PROGRAM SWProducts
(*SwenChen 2016.7.21 编辑为ＴＣ３*)
VAR
	fb_RecipeManCommands: 		RecipeManCommands;
	fbDirectoryCopy:			FB_DirectoryCopy;
	fbFileDelete:				FB_FileDelete;
	fbEnumFindFileEntry:		FB_EnumFindFileEntry;
	fbCreateDir:				FB_CreateDir;
	F_TRIGLOAD: 			F_TRIG;
	F_TRIGSave: 			F_TRIG;
	F_TRIGLOADFromUSB: 		F_TRIG;
	F_TRIGSaveToUSB: 		F_TRIG;
	F_TRIGDel: 				F_TRIG;
	F_TRIGYes: 				F_TRIG;
	F_TRIGNo: 				F_TRIG;
	TOF_File_load: 			TOF;
	stepLoad: 				INT;
	stepSave: 				INT;
	stepLoadFromUSB: 		INT;
	stepSaveToUSB: 			INT;
	stepDel: 					INT;
	stepInit: 					INT:=0;
	i:						INT;
	n: 						INT;
	j: 						INT;
	TimeCount:				INT;
	bInitState:				BOOL;
	bInit: 					BOOL:=TRUE;
	bInit_fbWritePersistentData: BOOL := TRUE;

	iLastSelIndex:			INT;
	TON_AutoReset: TON;
	DeviceNum: INT := 1;
	sDevice: STRING(INT#12);
	TON_WaitDone: TON;
END_VAR

DeviceNum:=1;	(*XP/CE操作系统选择*)

IF vbtLoad OR vbtSave THEN
	CASE DeviceNum OF
		1:(*xp*)
			sDevice:='C:\Products\';//不建议修改保存目录，其他地方也可能要改的
		2:(*usb*)
			;
		3:(*ce*)
			sDevice:='\Hard Disk\Products\';//不建议修改保存目录，其他地方也可能要改的
	END_CASE;
END_IF


IF NOT bInitState THEN
	Init();
ELSE
	IF ShowDiag THEN
		;//FB_FreePluse1s(tPluseCyle:=t#1s);
	END_IF
	F_TRIGYes(CLK:=vbtYes);
	F_TRIGNo(CLK:=vbtNo);
	HMISelect();
	ButtonDelet();
	ButtonLoad();
	ButtonSave();
	ButtonLoadFromUSB();
	ButtonSaveToUSB();
	ReflashFileList();
	if_data_change();
END_IF

ACTION ButtonDelet:
F_TRIGdel(CLK:=vbtdel );
CASE stepDel OF
	0:
		IF F_TRIGdel.Q THEN
			FOR i:=1 TO cnMaxRecepeNum DO
				IF vbtRecipeArr[i]=TRUE  AND strRecipeArr[i]<>'' THEN
					strShowDiagName:=strRecipeArr[i];
					ShowDiag:=TRUE;
					DiagIndex:=3;
					stepDel:=10;
					i:=1000;
					EXIT;
				END_IF
			END_FOR

		END_IF

	10:
		ShowDiag:=TRUE;
		IF F_TRIGYes.Q THEN
			ShowDiag:=FALSE;
			stepDel:=20;
		ELSIF F_TRIGNo.Q THEN
			ShowDiag:=FALSE;
			stepDel:=0;
		END_IF

	20:
		CASE DeviceNum OF
			1:(*xp*)
				fbFileDelete.sPathName:=CONCAT (CONCAT (sDevice , strShowDiagName),'.txtrecipe');
			2:(*usb*)
				;
			3:(*ce*)
				fbFileDelete.sPathName:=CONCAT (CONCAT (sDevice , strShowDiagName), '.txtrecipe');
		END_CASE;
		fbFileDelete
			(
			sNetId:='' ,
			ePath:=PATH_GENERIC ,
			bExecute:=TRUE ,
			tTimeout:=T#10s ,
			);
		IF NOT fbFileDelete.bBusy THEN
			fbFileDelete(bExecute:=FALSE);
			vbtFlash:=TRUE;
			stepDel:=30;
		END_IF

	30:
		IF NOT vbtFlash THEN
			FOR j:=1 TO cnMaxRecepeNum DO
				vbtRecipeArr[j]:=FALSE;
			END_FOR;
			stepDel:=0;
		END_IF

END_CASE
END_ACTION

ACTION ButtonLoad:
F_TRIGLOAD(CLK:=vbtLoad , Q=> );
CASE stepLoad OF
	0:
		IF F_TRIGLOAD.Q THEN
			FOR i:=1 TO cnMaxRecepeNum DO
				IF vbtRecipeArr[i]=TRUE  
				AND strRecipeArr[i]<>'' THEN
					strShowDiagName:=strRecipeArr[i];
					ShowDiag:=TRUE;
					DiagIndex:=1;
					stepLoad:=10;
					i:=1000;
					EXIT;
				END_IF
			END_FOR
		END_IF

	10:
		IF F_TRIGYes.Q THEN
			strCurrentReceipeName:=strShowDiagName;
			ShowDiag:=FALSE;
			TimeCount:=0;
			stepLoad:=20;
		ELSIF F_TRIGNo.Q THEN
			ShowDiag:=FALSE;
			stepLoad:=0;
		END_IF

	20:
	
		fb_RecipeManCommands.CreateRecipe
			(
			RecipeDefinitionName:=	'Recipes',
			RecipeName:=			'Test',
			);
		fb_RecipeManCommands.LoadFromAndWriteRecipe
			(
			RecipeDefinitionName:=	'Recipes',
			RecipeName:=			'Test',
			FileName:=				CONCAT(CONCAT(sDevice,strCurrentReceipeName),'.txtrecipe'),
			);
			stepLoad:=30;

	30:
		stepLoad:=40;

	40:
		stepLoad:=0;


END_CASE
END_ACTION

ACTION ButtonLoadFromUSB:
F_TRIGLOADFromUSB(CLK:=vbtLoadFromUSB , Q=> );
CASE stepLoadFromUSB OF
	0:
		IF F_TRIGLOADFromUSB.Q  AND NOT fbDirectoryCopy.bBusy THEN
			CASE DeviceNum OF
				1:(*xp*)
					fbDirectoryCopy.srcPathName:='C:\ProductsBackUp\';
					fbDirectoryCopy.destPathName:='C:\';
				2:(*usb*)
					;
				3:(*ce*)
					fbDirectoryCopy.srcPathName:='\Hard Disk2\';
					fbDirectoryCopy.destPathName:='\Hard Disk\';
			END_CASE
			strShowDiagName:='';
			DiagIndex:=7;
			stepLoadFromUSB:=10;
		END_IF

	10:
		ShowDiag:=TRUE;
		IF F_TRIGYes.Q THEN
			ShowDiag:=FALSE;
			stepLoadFromUSB:=20;
		ELSIF F_TRIGNo.Q THEN
			ShowDiag:=FALSE;
			stepLoadFromUSB:=30;
			vbtFlash:=TRUE;
		END_IF

	20:
		fbDirectoryCopy
			(
			srcNetId:='' ,
			DirectoryName:= 'Products',
			FileType:='XML' ,
			destNetId:='' ,
			bExecute:=TRUE,
			bFindFileList:=,
			tAdsTimeOut:=T#10s ,
			);
		IF fbDirectoryCopy.bBusy THEN
			IF  fbDirectoryCopy.bError AND  fbDirectoryCopy.nErrId=3 THEN
				fbDirectoryCopy.bContinueWhenErr:=F_TRIGYes.Q;
				fbDirectoryCopy.bCancelWhenErr:=F_TRIGNo.Q;
				strShowDiagName:=fbDirectoryCopy.srcFilesLists[fbDirectoryCopy.i].sFileName;
				ShowDiag:=TRUE;
				DiagIndex:=2;
			ELSE
				fbDirectoryCopy.bContinueWhenErr:=FALSE;
				fbDirectoryCopy.bCancelWhenErr:=FALSE;
				ShowDiag:=FALSE;
			END_IF
		ELSIF NOT fbDirectoryCopy.bBusy THEN
			stepLoadFromUSB:=21;
		END_IF

	21:
		IF  fbDirectoryCopy.bError AND  fbDirectoryCopy.nErrId=1 THEN
			strShowDiagName:='';
			ShowDiag:=TRUE;
			DiagIndex:=8;
			IF F_TRIGYes.Q OR F_TRIGNo.Q THEN
				fbDirectoryCopy(bExecute:=FALSE);
				ShowDiag:=FALSE;
				stepLoadFromUSB:=0;
			END_IF
		ELSE
			fbDirectoryCopy(bExecute:=FALSE);
			ShowDiag:=FALSE;
			stepLoadFromUSB:=30;
			vbtFlash:=TRUE;
		END_IF

	30:
		IF NOT vbtFlash THEN
			stepLoadFromUSB:=0;
		END_IF

END_CASE
END_ACTION

ACTION ButtonSave:
F_TRIGSAVE(CLK:=vbtSave , );

CASE stepSave OF
	0:
		IF F_TRIGSAVE.Q THEN
			IF strInputReceipeName='' THEN
				;
			ELSE
					FOR i:=1 TO cnMaxRecepeNum DO

							IF strRecipeArr[i]=strInputReceipeName THEN
								ShowDiag:=TRUE;
								DiagIndex:=2;
								stepSave:=10;
								strShowDiagName:=strRecipeArr[i];
								i:=1000;
							ELSIF strRecipeArr[i]='' THEN
								ShowDiag:=FALSE;
								stepSave:=20;
								i:=1000;
							END_IF;

					END_FOR;
			END_IF;
		END_IF;
	10:
		IF  F_TRIGYes.Q THEN
			ShowDiag:=FALSE;
			stepSave:=20;
		ELSIF  F_TRIGNo.Q THEN
			ShowDiag:=FALSE;
			stepSave:=0;
		END_IF;

	20:
		fb_RecipeManCommands.CreateRecipe
			(
			RecipeDefinitionName:=	'Recipes',
			RecipeName:=			'Prd',
			);
		fb_RecipeManCommands.ReadAndSaveRecipeAs		
			(
			RecipeDefinitionName:=	'Recipes',
			RecipeName:=			'Prd',
			FileName:=				CONCAT(CONCAT(sDevice,strInputReceipeName),'.txtrecipe'),
			);	
		stepSave:=30;

		
	30:
		TON_WaitDone(IN:=TRUE , PT:=T#500MS );
		IF TON_WaitDone.Q THEN
			TON_WaitDone(IN:=FALSE);
			vbtFlash:=TRUE;
			stepSave:=40;
		END_IF
	40:
		IF NOT vbtFlash THEN
			stepSave:=0;
		END_IF

END_CASE;
END_ACTION

ACTION ButtonSaveToUSB:
F_TRIGSaveToUSB(CLK:=vbtSaveToUSB , Q=> );
CASE stepSaveToUSB OF
	0:
		IF F_TRIGSaveToUSB.Q  AND NOT fbDirectoryCopy.bBusy THEN
			CASE DeviceNum OF
				1:(*xp*)
					fbDirectoryCopy.srcPathName:='C:\';
					fbDirectoryCopy.destPathName:='C:\ProductsBackUp\';
				2:(*usb*)
					;
				3:(*ce*)
					fbDirectoryCopy.srcPathName:='\Hard Disk\';
					fbDirectoryCopy.destPathName:='\Hard Disk2\';
			END_CASE;
			strShowDiagName:='';
			DiagIndex:=6;
			stepSaveToUSB:=10;
		END_IF

	10:
		ShowDiag:=TRUE;
		IF F_TRIGYes.Q THEN
			ShowDiag:=FALSE;
			stepSaveToUSB:=20;
		ELSIF F_TRIGNo.Q THEN
			ShowDiag:=FALSE;
			stepSaveToUSB:=0;
		END_IF

	20:
		fbDirectoryCopy
			(
			srcNetId:='' ,
			DirectoryName:= 'Products',
			FileType:='XML' ,
			destNetId:='' ,
			bExecute:=TRUE,
			bFindFileList:=,
			tAdsTimeOut:=T#10s ,
			);
		IF fbDirectoryCopy.bBusy THEN
			IF  fbDirectoryCopy.bError AND  fbDirectoryCopy.nErrId=3 THEN
				fbDirectoryCopy.bContinueWhenErr:=F_TRIGYes.Q;
				fbDirectoryCopy.bCancelWhenErr:=F_TRIGNo.Q;
				strShowDiagName:=fbDirectoryCopy.srcFilesLists[fbDirectoryCopy.i].sFileName;
				ShowDiag:=TRUE;
				DiagIndex:=2;
			ELSE
				fbDirectoryCopy.bContinueWhenErr:=FALSE;
				fbDirectoryCopy.bCancelWhenErr:=FALSE;
				ShowDiag:=FALSE;
			END_IF
		ELSIF NOT fbDirectoryCopy.bBusy THEN
			fbDirectoryCopy(bExecute:=FALSE);
			ShowDiag:=FALSE;
			stepSaveToUSB:=0;
		END_IF


END_CASE
END_ACTION

ACTION HMISelect:
FOR i:=1 TO (cnMaxRecepeNum-1) DO
	IF strRecipeArr[i]='' AND strRecipeArr[(i+1)]<>'' THEN
		strRecipeArr[i]:=strRecipeArr[(i+1)];
		strRecipeArr[(i+1)]:='';
	END_IF;
END_FOR;


IF iLastSelIndex <> iSelectIndex THEN
	iLastSelIndex := iSelectIndex;
	IF iSelectIndex>=1
	AND iSelectIndex<=cnMaxRecepeNum THEN
		FOR i:=1 TO cnMaxRecepeNum DO
			IF strRecipeArr[i]<>'' THEN
					IF i=iSelectIndex THEN
						strInputReceipeName:=strRecipeArr[i];
						vbtRecipeArr[i]:=TRUE;
					ELSE
						vbtRecipeArr[i]:=FALSE;
					END_IF
			ELSE
				vbtRecipeArr[i]:=FALSE;
			END_IF
		END_FOR
	END_IF
END_IF
END_ACTION

ACTION if_data_change:

;
END_ACTION

ACTION Init:
(*
ReflashFileList();
IF NOT vbtFlash THEN
	bInitState:=TRUE;
END_IF
*)


CASE stepInit OF

	0:	(*CheckDeviceName*)
		CASE DeviceNum OF
			1:(*xp*)
				fbEnumFindFileEntry.sPathName:=
				fbCreateDir.sPathName:='C:\Products';
			2:(*usb*)
					;
			3:(*ce*)
				fbEnumFindFileEntry.sPathName:=
				fbCreateDir.sPathName:='\Hard Disk\Products';
		END_CASE
		fbEnumFindFileEntry
			(
			sNetId:='' , 
			(*sPathName:=CONCAT(srcPathName,DirectoryName),*)
			eCmd:=eEnumCmd_First ,
			bExecute:=TRUE ,
			tTimeout:=T#10s ,
			);
		IF NOT  fbEnumFindFileEntry.bBusy THEN
			IF NOT  fbEnumFindFileEntry.bEOE THEN		(*target dir is exist*)
				vbtFlash:=TRUE;
				stepInit:=20;
			ELSE
				stepInit:=10;
			END_IF
			fbEnumFindFileEntry(bExecute:=FALSE);
			vbtLoad:=TRUE;
		END_IF

	10:	(*createt dir  *)
		fbCreateDir
			(
			sNetId:='',
			(*sPathName:= CONCAT(destPathName,DirectoryName),*)
			ePath:= PATH_GENERIC,
			bExecute:=TRUE,
			tTimeout:=t#10s
			);
		IF NOT fbCreateDir.bBusy THEN
			fbCreateDir(bExecute:=FALSE);
			stepInit:=30;
		END_IF

	20:	(*ReflashFileList*)
		ReflashFileList();
		IF NOT vbtFlash THEN
			IF strCurrentReceipeName<>'' THEN
				FOR i:=1 TO cnMaxRecepeNum DO
					IF strRecipeArr[i]=strCurrentReceipeName THEN
						stepInit:=30;
						EXIT;
					END_IF
				END_FOR
				IF i> cnMaxRecepeNum THEN
					stepInit:=40;
				END_IF
			ELSE
				stepInit:=40;
			END_IF
		END_IF

	30:	(*loadParameters*)
		stepInit:=40;

	40:	(*InitFinish*)
		bInitState:=TRUE;


END_CASE
END_ACTION

ACTION ReflashFileList:
IF vbtFlash THEN
		CASE DeviceNum OF
			1:(*xp*)
				fbDirectoryCopy.srcPathName:='C:\';
			2:(*usb*)
				;
			3:(*ce*)
				fbDirectoryCopy.srcPathName:='\Hard Disk\';
		END_CASE;
		fbDirectoryCopy
			(
			srcNetId:='' ,
			DirectoryName:= 'Products',
			FileType:='txtrecipe' ,
			bFindFileList:=TRUE,
			tAdsTimeOut:=T#10s ,
			);
		IF NOT fbDirectoryCopy.bBusy THEN
			fbDirectoryCopy(bFindFileList:=FALSE);
			FOR i:=1 TO cnMaxRecepeNum DO
				strRecipeArr[i]:=LEFT(fbDirectoryCopy.srcFilesLists[i].sFileName, (LEN(fbDirectoryCopy.srcFilesLists[i].sFileName) - 10));
			END_FOR
			vbtFlash:=FALSE;;
		END_IF
END_IF
END_ACTION

END_PROGRAM
